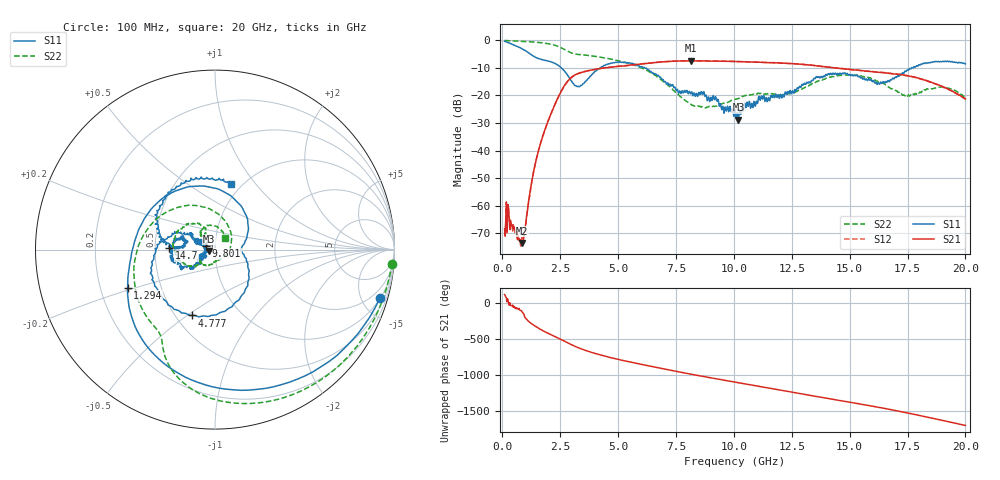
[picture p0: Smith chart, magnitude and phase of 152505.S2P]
!  2-Port S-parameters saved by WinCal
! VAR MeasName=S-Parameters (CALIBRATED_DATA) read from VNA (N5230C)
! VAR MeasDate=4/10/2015 9:27:57 AM
! VAR NAME=152505
! VAR FILENAME=152505.S2P
! VAR DATE=4/10/2015 9:27:57 AM
! VAR PHYS_PORTS=1,2
# Hz S DB R 50
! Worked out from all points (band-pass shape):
!   801 points, 100 MHz to 20 GHz, reference 50 ohm
!   highest |S21| = -7.46 dB at 8.159 GHz (marker M1); lowest = -73.5 dB at 846.2 MHz (marker M2)
!   |S21| within 3 dB of the highest: 4.094 GHz to 14.87 GHz (10.78 GHz wide, 114 % of centre)
!   lowest |S11| = -28.8 dB at 10.2 GHz (marker M3), VSWR 1.08, Z = 46.6 - j0.648 ohm
!   |S11| at or under -10 dB: 2.548 GHz to 4.243 GHz (1.694 GHz wide, 49.9 % of centre); 6.148 GHz to 17.68 GHz (11.53 GHz wide, 96.8 % of centre); 17.72115 GHz to 17.74525 GHz (24.1 MHz wide, 0.136 % of centre)
!   |S22| runs from -24.6 to -0.1 dB; largest |S21 - S12| = 0.0069
!   S11 on the Smith chart (normalised r, x): 100 MHz: 1.03, -6.81; 1.294 GHz: 0.32, -0.19; 4.777 GHz: 0.60, -0.52; 9.801 GHz: 0.90, +0.04; 14.7 GHz: 0.59, +0.01; 20 GHz: 0.89, +0.76
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1e8  -0.37 -16.3  -68.32 119.7  -69.72 120.5  -0.08 -4.6
2.74125e8  -0.92 -41.0  -61.52 -8.5  -61.71 -7.4  -0.17 -11.5
4.73125e8  -1.61 -67.1  -68.07 -55.3  -66.85 -55.5  -0.25 -19.4
8.4625e8  -3.06 -111.7  -73.54 -114.9  -71.54 -116.3  -0.38 -34.3
1.294e9  -5.49 -156.4  -50.29 69.1  -50.26 69.2  -0.61 -52.5
1.716875e9  -7.04 170.9  -35.59 -15.9  -35.54 -15.9  -0.94 -70.4
2.363625e9  -8.82 101.6  -21.59 -116.5  -21.58 -116.6  -2.08 -99.7
2.910875e9  -13.89 26.4  -14.05 155.9  -14.06 156.1  -4.34 -118.8
3.43325e9  -16.32 -6.5  -11.64 82.6  -11.62 83.0  -5.29 -129.1
4.7765e9  -8.20 -109.6  -9.69 -43.1  -9.64 -42.9  -7.01 -173.9
5.672e9  -8.62 -162.8  -8.92 -107.0  -8.87 -107.2  -8.95 148.3
6.741625e9  -12.75 154.5  -7.97 -176.9  -7.96 -177.3  -13.50 90.1
8.1595e9  -18.92 156.9  -7.46 94.2  -7.45 94.1  -23.28 -24.3
9.80125e9  -25.27 157.3  -7.66 -1.5  -7.65 -1.4  -22.27 -100.3
1.005e10  -25.33 -171.0  -7.69 -15.9  -7.71 -16.0  -21.39 -103.5
1.019925e10  -28.82 -168.9  -7.74 -24.4  -7.77 -24.2  -21.15 -109.4
1.159225e10  -20.15 -157.4  -8.17 -102.3  -8.08 -102.7  -19.43 -140.3
1.338325e10  -14.60 -147.3  -9.11 155.5  -9.05 155.7  -15.73 -145.4
1.470162e10  -11.89 178.1  -10.34 82.2  -10.29 81.0  -12.62 175.2
1.669162e10  -14.93 177.5  -11.97 -31.8  -11.98 -32.9  -17.05 116.9
1.828362e10  -8.27 146.2  -14.55 -137.3  -14.48 -137.4  -18.07 130.1
2e10  -8.52 76.2  -21.28 102.9  -21.37 103.2  -21.19 48.1
